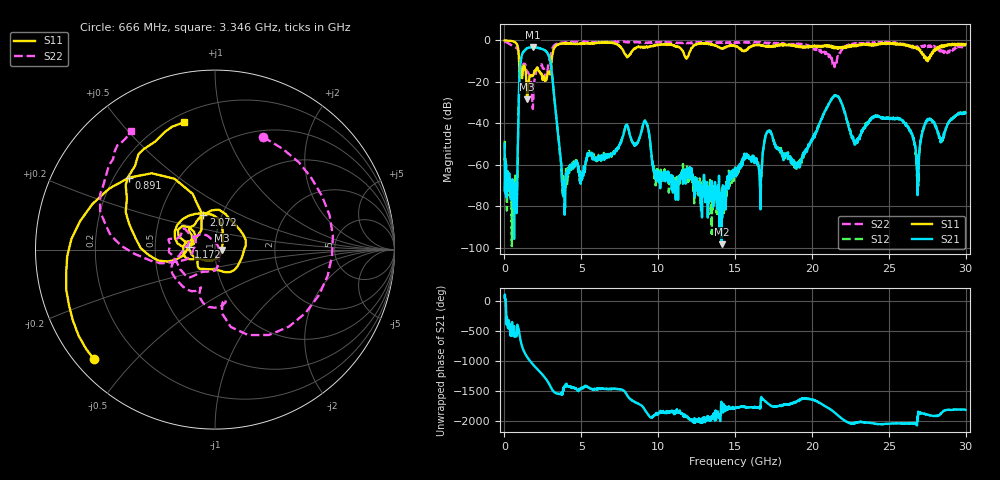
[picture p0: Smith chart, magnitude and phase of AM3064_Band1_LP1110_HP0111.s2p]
# Hz S DB R 50.0
!freq dBS11 angS11 dBS21 angS21 dBS12 angS12 dBS22 angS22
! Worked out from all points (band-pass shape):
!   1600 points, 10 MHz to 29.98 GHz, reference 50 ohm
!   highest |S21| = -3.25 dB at 1.828 GHz (marker M1); lowest = -98.4 dB at 14.12 GHz (marker M2)
!   |S21| within 3 dB of the highest: 1.177 GHz to 2.806 GHz (1.629 GHz wide, 81.8 % of centre)
!   lowest |S11| = -28.4 dB at 1.472 GHz (marker M3), VSWR 1.08, Z = 54 - j0.248 ohm
!   |S11| at or under -10 dB: 949.7 MHz to 3.063 GHz (2.114 GHz wide, 105 % of centre); 27.52538 GHz to 27.52996 GHz (4.586 MHz wide, 0.0167 % of centre)
!   |S22| runs from -33.1 to -0.4 dB; largest |S21 - S12| = 0.0087
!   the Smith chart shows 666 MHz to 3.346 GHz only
!   S11 on the Smith chart (normalised r, x): 666 MHz: 0.05, -0.38; 891 MHz: 0.26, +0.34; 1.172 GHz: 0.74, +0.02; 2.072 GHz: 0.82, +0.33; 3.346 GHz: 0.25, +0.76
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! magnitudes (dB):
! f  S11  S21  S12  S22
! 10 MHz  0.0  -50.0  -48.5  -0.4
! 666 MHz  -0.8  -72.2  -76.1  -3.3
! 891 MHz  -4.1  -42.8  -42.6  -5.0
! 1.172 GHz  -16.7  -6.3  -6.2  -12.9
! 1.472 GHz  -28.4  -3.8  -3.8  -15.0
! 1.828 GHz  -16.9  -3.3  -3.2  -32.3
! 2.072 GHz  -13.8  -3.5  -3.5  -14.2
! 2.897 GHz  -15.1  -7.8  -7.7  -10.0
! 3.346 GHz  -2.7  -35.2  -35.4  -1.9
! 3.871 GHz  -1.4  -73.1  -66.0  -1.1
! 5.015 GHz  -1.5  -66.2  -64.8  -0.7
! 9.157 GHz  -3.4  -39.1  -38.8  -1.1
! 10 GHz  -2.2  -63.8  -63.7  -0.9
! 14.12 GHz  -3.9  -98.4  -82.3  -1.1
! 15 GHz  -2.7  -62.3  -61.4  -1.3
! 19.99 GHz  -3.2  -48.4  -47.7  -3.1
! 21.51 GHz  -3.1  -26.9  -26.8  -11.2
! 22.8 GHz  -2.2  -50.1  -50.1  -2.0
! 25 GHz  -1.2  -37.5  -37.6  -1.1
! 26.87 GHz  -4.2  -74.7  -62.8  -3.0
! 27.51 GHz  -9.2  -38.6  -38.2  -3.1
! 29.98 GHz  -1.8  -34.9  -35.1  -2.8
